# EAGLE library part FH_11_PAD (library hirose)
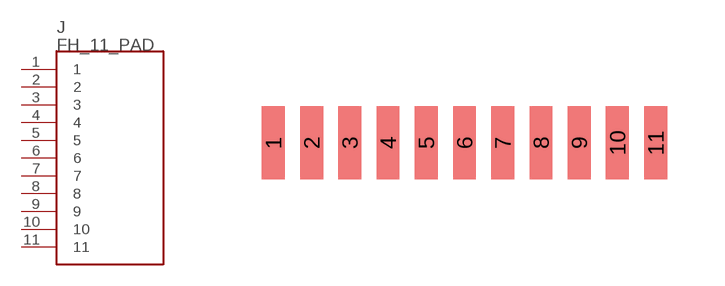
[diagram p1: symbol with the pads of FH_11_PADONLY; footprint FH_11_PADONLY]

Designator prefix J

## FH_11_PAD  [FH_11_PADONLY]
1  1
2  2
3  3
4  4
5  5
6  6
7  7
8  8
9  9
10  10
11  11

## Footprint FH_11_PADONLY (pad centres in mm)
smd 0.6 x 1.9: 1 -5,-0.62; 2 -4,-0.62; 3 -3,-0.62; 4 -2,-0.62; 5 -1,-0.62; 6 0,-0.62; 7 1,-0.62; 8 2,-0.62; 9 3,-0.62; 10 4,-0.62; 11 5,-0.62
